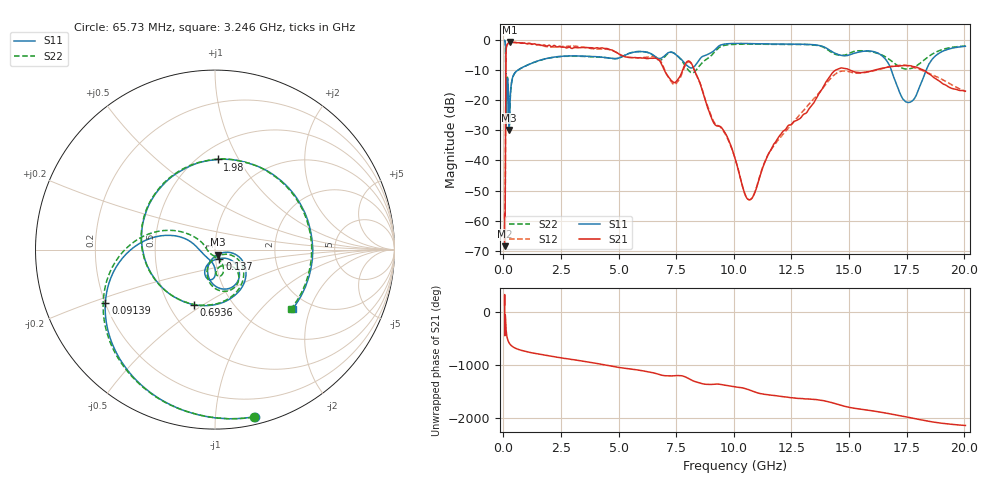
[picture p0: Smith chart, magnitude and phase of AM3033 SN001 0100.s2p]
# Hz S DB R 50
!freq MagS11 AngS11 MagS21 AngS21 MagS12 AngS12 MagS22 AngS22
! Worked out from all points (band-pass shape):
!   1601 points, 50 MHz to 20.05 GHz, reference 50 ohm
!   highest |S21| = -0.70 dB at 295.2 MHz (marker M1); lowest = -68.5 dB at 64.51 MHz (marker M2)
!   |S21| within 3 dB of the highest: 112.4 MHz to 4.793 GHz (4.68 GHz wide, 191 % of centre)
!   lowest |S11| = -29.9 dB at 253.2 MHz (marker M3), VSWR 1.07, Z = 51.4 - j2.9 ohm
!   |S11| at or under -10 dB: 97.39 MHz to 626.8 MHz (529.4 MHz wide, 146 % of centre); 16.83 GHz to 18.35 GHz (1.514 GHz wide, 8.61 % of centre)
!   |S22| runs from -29.6 to -0.2 dB; largest |S21 - S12| = 0.063
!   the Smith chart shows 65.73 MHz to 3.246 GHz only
!   S11 on the Smith chart (normalised r, x): 65.73 MHz: 0.06, -1.27; 91.39 MHz: 0.20, -0.22; 137 MHz: 1.04, -0.11; 693.6 MHz: 0.66, -0.46; 1.98 GHz: 0.61, +0.82; 3.246 GHz: 1.63, -1.53
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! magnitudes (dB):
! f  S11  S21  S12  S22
! 50 MHz  -0.2  -57.9  -61.6  -0.2
! 64.51 MHz  -0.3  -68.5  -66.4  -0.3
! 65.73 MHz  -0.4  -67.3  -65.0  -0.4
! 91.39 MHz  -3.4  -21.9  -21.9  -3.4
! 105.4 MHz  -23.6  -5.2  -5.2  -29.5
! 135.9 MHz  -25.3  -2.0  -2.0  -20.1
! 137 MHz  -25.1  -2.0  -2.0  -19.9
! 180 MHz  -12.9  -1.3  -1.4  -12.5
! 253.2 MHz  -29.9  -0.7  -0.8  -28.0
! 295.2 MHz  -19.1  -0.7  -0.7  -19.4
! 369.6 MHz  -13.3  -0.8  -0.7  -13.5
! 693.6 MHz  -9.7  -0.9  -1.0  -9.7
! 1.005 GHz  -8.5  -1.3  -1.1  -8.4
! 1.98 GHz  -6.0  -1.7  -2.3  -6.0
! 2.722 GHz  -5.3  -2.6  -2.2  -5.4
! 3.246 GHz  -5.3  -2.6  -2.1  -5.4
! 7.402 GHz  -4.4  -14.1  -14.8  -4.4
! 8.251 GHz  -9.0  -9.3  -9.4  -10.8
! 10.69 GHz  -1.2  -53.0  -53.1  -1.4
! 14.53 GHz  -4.8  -9.6  -10.8  -5.0
! 17.59 GHz  -20.7  -8.5  -8.6  -9.6
! 20.05 GHz  -2.1  -17.0  -17.0  -2.0
